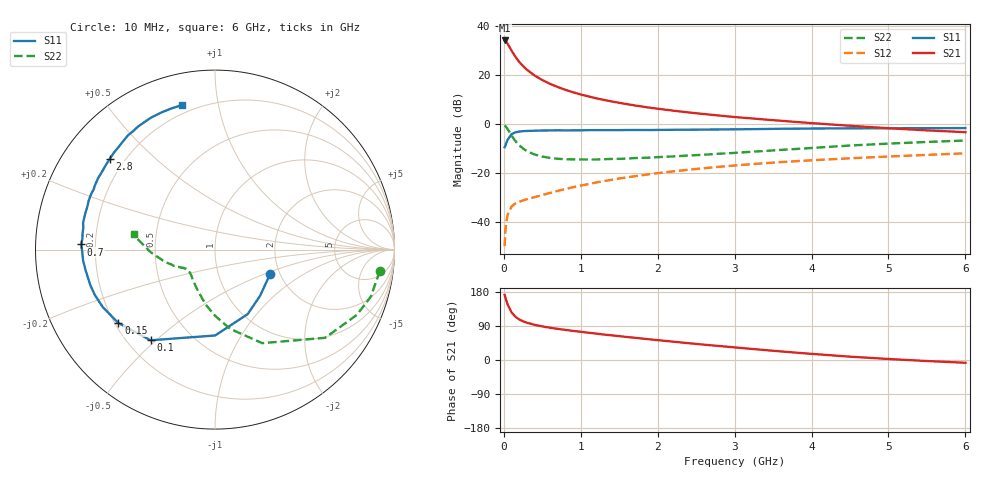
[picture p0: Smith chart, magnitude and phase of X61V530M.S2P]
! SIEMENS Small Signal Semiconductors
! BFP193W
! Si NPN RF Bipolar Junction Transistor in SOT343
! VCE = 1.5 V  IC = 30 mA
! Common Emitter S-Parameters:  April 1994
# GHz  S  MA  R  50
!  f  S11  S21  S12  S22
! GHz  MAG  ANG  MAG  ANG  MAG  ANG  MAG  ANG
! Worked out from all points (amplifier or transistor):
!   40 points, 10 MHz to 6 GHz, reference 50 ohm
!   highest |S21| = 34.1 dB at 10 MHz (marker M1)
!   |S21| within 3 dB of that: start of sweep to 79.37 MHz
!   unconditionally stable (mu >= 1): 720.5 MHz to 4.195 GHz
!   at 200 MHz: K = 0.47, MSG = 28.6 dB, |S12| = -31.8 dB
!   at 1.5 GHz: K = 1.15, MAG = 13.1 dB, |S12| = -22.2 dB
!   at 6 GHz: K = 0.95, MSG = 4.3 dB, |S12| = -12.0 dB
!   S11 on the Smith chart (normalised r, x): 10 MHz: 1.78, -0.54; 100 MHz: 0.29, -0.48; 150 MHz: 0.21, -0.32; 700 MHz: 0.15, +0.02; 2.8 GHz: 0.14, +0.37; 6 GHz: 0.15, +0.78
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0.01  0.3358 -23.7  50.93 171.7  0.0032 81.0  0.9258 -7.5
0.02  0.3597 -45.7  49.95 165.2  0.0067 76.2  0.907 -16.8
0.03  0.4029 -63.1  48.27 158.3  0.0096 72.6  0.8701 -24.7
0.05  0.4785 -89.9  43.38 146.1  0.0142 61.7  0.7861 -38.7
0.1  0.6198 -125.4  31.66 125.9  0.0206 47.4  0.584 -63.2
0.15  0.6762 -142.8  23.7 114.1  0.0239 42.2  0.4494 -79.2
0.2  0.7025 -152.8  18.61 107.0  0.0258 40.5  0.3677 -90.1
0.25  0.7156 -159.3  15.29 102.0  0.0275 40.6  0.3166 -98.4
0.3  0.7222 -163.9  12.85 98.4  0.0292 41.6  0.279 -105.2
0.4  0.7299 -170.8  9.795 92.8  0.0321 44.2  0.2386 -115.3
0.5  0.7376 -175.4  7.904 88.6  0.0356 47.7  0.2167 -122.8
0.6  0.7394 -178.9  6.61 85.1  0.0391 49.8  0.2033 -128.6
0.7  0.7458 177.8  5.716 82.2  0.0431 51.8  0.1952 -132.7
0.9  0.7436 172.8  4.453 76.8  0.0513 54.9  0.1898 -138.5
1.1  0.7496 168.6  3.668 72.0  0.0593 56.8  0.1882 -142.5
1.6  0.7544 159.1  2.552 60.7  0.0814 58.1  0.1969 -147.8
2.2  0.7632 148.7  1.877 48.4  0.1079 56.3  0.2182 -153.4
2.8  0.7745 139.1  1.49 36.9  0.1338 53.0  0.2476 -158.7
3.2  0.7846 133.2  1.311 29.7  0.1505 50.4  0.2698 -163.3
4.5  0.8172 115.9  0.921 8.8  0.1995 41.0  0.3637 -178.4
5.5  0.823 107.3  0.742 -2.7  0.2343 34.3  0.4302 172.7
6  0.8262 103.0  0.682 -7.3  0.2524 31.3  0.4605 169.2
